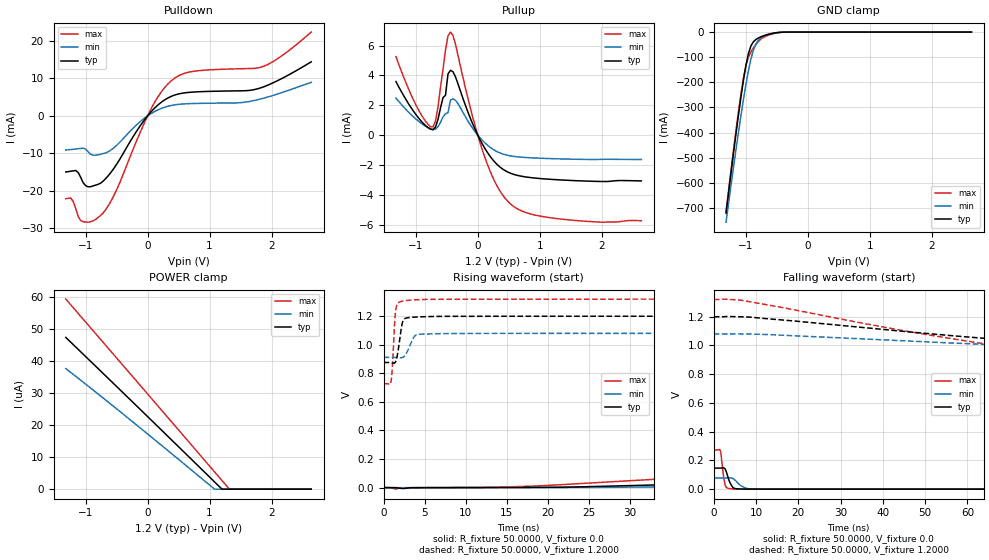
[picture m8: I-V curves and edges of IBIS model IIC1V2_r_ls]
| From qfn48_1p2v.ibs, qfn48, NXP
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[Model] IIC1V2_r_ls
|   Model IIC1V2_r_ls
| This model was characterised for following simulation conditions:
| External (pad) voltage:
|   - Typ: 1.2V,   - Min: 1.08V,   - Max: 1.32V
| Library cells for typ/min/max conditions are connected as defined below:
|  IO - External Pad
|  A - Core Input
|  EN - Output Buffer Enable
|  BOOST - vdde
|  EGP - vdd
|  EHS - gnd
|  ENZI - vdd
|  EPD - vdd
|  EPUN - gnd
|  ZI - NC
|  ZIF - NC
|  gnd - gnd
|  gnde - gnde
|  vdd - vdd
|  vdde - vdde
| All other pins connected to ground
Model_type I/O
Polarity   Non-Inverting
Enable   Active-Low
Vinl =   0.5400V
Vinh =   1.2600V
Vmeas =  0.9000V
Cref =   0.0F
Rref =   1.0000k
Vref =   0.0V
C_comp   3.6164pF   3.4768pF   3.7417pF
|C_comp_pullup   0.9402pF   0.8991pF   0.9548pF
|C_comp_pulldown   2.3240pF   2.4771pF   2.1787pF
[Model Spec]
| variable   typ   min   max
Vinh   0.3600V   0.3240V   0.3960V
Vinl   0.8400V   0.7560V   0.9240V
Vmeas   0.6000V   0.5400V   0.6600V
[Temperature Range]   25.0000   0.1250k   -40.0000
[Voltage Range]   1.2000V   1.0800V   1.3200V
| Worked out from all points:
|   slope of the pulldown table from 0 to 0.18 V, typ, clamps not added: 58.3 ohm
|   slope of the pullup table from 0 to 0.18 V, typ, clamps not added: 138 ohm
|   GND clamp passes 1 mA (typ) near -0.45 V on its own axis
|   rising waveform, R_fixture 50.0000, V_fixture 0.0: 20-80 % time 73.3ns typ, 82.8ns min, 61.7ns max; typ from 0 V to 0.146 V
|   rising waveform, R_fixture 50.0000, V_fixture 1.2000: 20-80 % time 495ps typ, 789ps min, 329ps max; typ from 0.876 V to 1.2 V
|   falling waveform, R_fixture 50.0000, V_fixture 0.0: 20-80 % time 1.12ns typ, 1.9ns min, 699ps max; typ from 0.146 V to 0 V
|   falling waveform, R_fixture 50.0000, V_fixture 1.2000: 20-80 % time 83.2ns typ, 98.8ns min, 62.6ns max; typ from 1.2 V to 0.876 V
[Pulldown]
|Voltage   I(typ)   I(min)   I(max)
-1.32V    -14.96mA   -9.099mA   -22.09mA
-1.24V    -14.75mA   -8.982mA   -21.89mA
-1.16V    -14.56mA   -8.83mA    -24.7mA
-1.04V    -17.82mA   -8.609mA   -28.21mA
-920mV    -18.88mA   -10.21mA   -28.21mA
-720mV    -17.44mA   -10.07mA   -25.94mA
-520mV    -13.41mA   -8.157mA   -20.44mA
80mV      1.521mA    840uA      2.628mA
440mV     5.569mA    2.951mA    10.1mA
760mV     6.377mA    3.307mA    11.92mA
1.84V     7.555mA    4.581mA    13.06mA
2.64V     14.41mA    8.944mA    22.34mA
[Pullup]
|Voltage   I(typ)   I(min)   I(max)
-1.32V    3.586mA    2.482mA    5.256mA
-960mV    1.175mA    947.4uA    1.725mA
-720mV    361.5uA    375.5uA    554.5uA
-640mV    1.072mA    568.3uA    1.915mA
-520mV    2.67mA     1.432mA    5.707mA
-480mV    4.094mA    1.5mA      6.648mA
-440mV    4.341mA    2.344mA    6.901mA
120mV     -924.8uA   -536.9uA   -1.554mA
360mV     -2.143mA   -1.197mA   -3.751mA
600mV     -2.653mA   -1.434mA   -4.838mA
1.4V      -3.016mA   -1.6mA     -5.648mA
2.64V     -3.069mA   -1.636mA   -5.736mA
[GND_clamp]
|Voltage   I(typ)   I(min)   I(max)
-1.32V    -720.7mA   -756.5mA   -713.8mA
-1.12V    -330.9mA   -399.5mA   -316.8mA
-1.04V    -192.4mA   -269.2mA   -184.4mA
-1V       -133.6mA   -209.3mA   -133.5mA
-960mV    -86.74mA   -154.7mA   -99.46mA
-920mV    -55.69mA   -108.2mA   -79.02mA
-880mV    -39.02mA   -72.35mA   -63.71mA
-840mV    -29.9mA    -48mA      -50.26mA
-760mV    -18.93mA   -23.39mA   -28.32mA
-640mV    -9.22mA    -8.628mA   -12.73mA
-400mV    -335.3uA   -402.3uA   -442.6uA
2.64V     0A         0A         0A
[POWER_clamp]
|Voltage   I(typ)   I(min)   I(max)
-1.32V    47.4uA     37.67uA    59.39uA
-280mV    27.94uA    21.65uA    36.04uA
1.08V     2.274uA    0A         5.413uA
1.2V      0A         0A         2.707uA
1.32V     0A         0A         0A
2.64V     0A         0A         0A
[Ramp]
| variable   typ   min   max
dV/dt_r  87.6550m/73.3048n   46.3571m/82.8164n   0.1635/61.7281n
dV/dt_f  0.1940/83.1773n   0.1007/98.8308n   0.3551/62.5986n
R_load = 50.0000
[Rising Waveform]
R_fixture= 50.0000
V_fixture= 0.0
V_fixture_min= 0.0
V_fixture_max= 0.0
|time   V(typ)   V(min)   V(max)
0s        642.2pV    57.99nV    36.63pV
1.473ns   -824.5uV   129.6uV    -10.9mV
2.402ns   -6.553mV   -429.4uV   -648.4uV
17.9ns    1.109mV    285.7uV    9.858mV
56.7ns    53.85mV    21.65mV    132.8mV
94.33ns   99.86mV    45.75mV    219.2mV
113.2ns   116.5mV    55.08mV    245.8mV
143.9ns   133.7mV    65.8mV     264.1mV
250.2ns   145.5mV    76.33mV    272.2mV
1us       146.1mV    77.26mV    272.4mV
[Rising Waveform]
R_fixture= 50.0000
V_fixture= 1.2000
V_fixture_min= 1.0800
V_fixture_max= 1.3200
|time   V(typ)   V(min)   V(max)
0s        875.8mV    911.4mV    727.2mV
904.3ps   874mV      911.7mV    743.4mV
1.064ns   871.8mV    911.6mV    845.5mV
1.399ns   875.1mV    910.5mV    1.206V
1.675ns   927.2mV    909.2mV    1.286V
2.173ns   1.123V     908.3mV    1.303V
2.476ns   1.177V     917mV      1.306V
3.885ns   1.193V     1.065V     1.314V
6.209ns   1.197V     1.076V     1.318V
1us       1.199V     1.079V     1.319V
[Falling Waveform]
R_fixture= 50.0000
V_fixture= 0.0
V_fixture_min= 0.0
V_fixture_max= 0.0
|time   V(typ)   V(min)   V(max)
0s        146.1mV    77.29mV    272.5mV
1.553ns   146.3mV    77.3mV     267.1mV
1.752ns   147mV      77.28mV    233.1mV
2.289ns   148.7mV    77.22mV    93.37mV
2.868ns   128.8mV    77.74mV    16.48mV
4.289ns   21.84mV    76.78mV    1.938mV
5.798ns   1.845mV    39.79mV    661.4uV
7.983ns   431.6uV    3.788mV    432.4uV
12.4ns    257.8uV    259.1uV    243.4uV
1us       25.86nV    100.8nV    14.91nV
[Falling Waveform]
R_fixture= 50.0000
V_fixture= 1.2000
V_fixture_min= 1.0800
V_fixture_max= 1.3200
|time   V(typ)   V(min)   V(max)
0s        1.199V     1.079V     1.319V
6.707ns   1.199V     1.08V      1.313V
41.97ns   1.106V     1.036V     1.118V
67.75ns   1.041V     1.003V     994mV
97.27ns   979mV      972.7mV    808.6mV
111.9ns   947.2mV    960.6mV    767.4mV
134.8ns   906.4mV    944.6mV    741.5mV
176.6ns   881.8mV    925mV      730.2mV
265.6ns   876.6mV    913.3mV    727.7mV
1us       875.9mV    911.5mV    727.2mV
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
